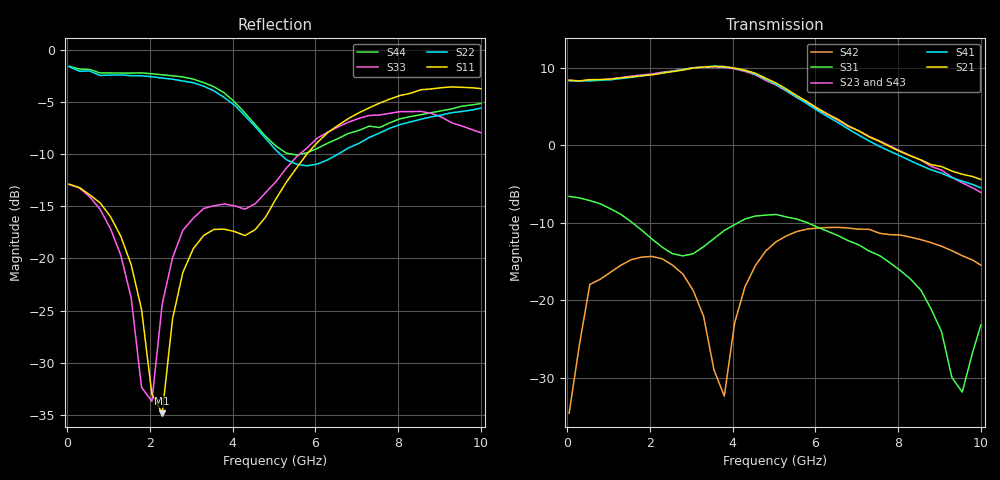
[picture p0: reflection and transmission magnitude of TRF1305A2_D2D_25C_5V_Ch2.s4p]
!Created with skrf (http://scikit-rf.org).
# Hz S MA R 50.0
! PORT[1] = INP
! PORT[2] = OUTM
! PORT[3] = INM
! PORT[4] = OUTP
!freq magS11 angS11 magS12 angS12 magS13 angS13
! magS14 angS14
! magS21 angS21 magS22 angS22 magS23 angS23
! magS24 angS24
! magS31 angS31 magS32 angS32 magS33 angS33
! magS34 angS34
! magS41 angS41 magS42 angS42 magS43 angS43
! magS44 angS44
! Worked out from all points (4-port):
!   41 points, 50 MHz to 10 GHz, reference 50 ohm
!   strongest paths, dB at 50 MHz, 2.55 GHz, 5.05 GHz, 7.55 GHz, 10 GHz:
!     S21: 8.4, 9.5, 8.0, 0.5, -4.4
!     S41: 8.3, 9.5, 7.8, -0.2, -5.5
!     S23: 8.4, 9.6, 7.7, 0.5, -6.1
!     S43: 8.3, 9.5, 7.7, 0.4, -5.9
!     S31: -6.6, -14.0, -9.0, -14.3, -23.2
!     S42: -34.6, -15.5, -12.5, -11.4, -15.5
!   lowest |S11| = -34.8 dB at 2.3 GHz (marker M1), VSWR 1.04, Z = 51.2 + j1.41 ohm
!   |S11| at or under -10 dB: start of sweep to 5.795 GHz
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5e7  0.2266 -3.3  0.00462 54.8  0.4625 -2.6  0.003948 133.1
     2.618 177.2  0.8278 177.5  2.617 -2.4  0.02086 122.0
     0.4668 -3.0  0.004925 134.3  0.2257 -2.3  0.005425 -2.4
     2.593 -2.6  0.01859 127.6  2.592 177.6  0.8326 177.6
2.3e9  0.0181 49.3  0.04119 -35.9  0.2165 -129.9  0.02643 -63.0
       2.911 63.0  0.7302 101.4  2.951 -117.4  0.183 -16.7
       0.2193 -128.6  0.02765 -64.5  0.06053 75.2  0.03866 -33.2
       2.923 -114.5  0.1845 -15.0  2.911 62.3  0.7569 99.3
3.55e9  0.1376 27.0  0.05256 -79.4  0.2484 114.8  0.02407 -130.3
        3.215 -11.6  0.6344 59.3  3.189 166.5  0.0283 -111.0
        0.2491 116.3  0.02722 -131.9  0.1786 35.4  0.05021 -79.5
        3.228 170.3  0.0355 -93.2  3.17 -13.3  0.6632 57.2
4.55e9  0.1375 30.0  0.05845 -120.0  0.3406 56.4  0.01795 -175.7
        2.906 -78.4  0.4267 32.8  2.838 98.9  0.1819 65.6
        0.3484 58.4  0.02007 172.8  0.1828 34.1  0.05493 -122.4
        2.868 103.3  0.1667 70.0  2.82 -80.4  0.4362 32.7
5.8e9  0.3172 22.9  0.05704 -169.0  0.3059 11.5  0.008715 164.8
       1.908 -153.5  0.2776 41.7  1.873 23.7  0.2854 13.9
       0.3163 11.6  0.01159 136.3  0.3383 22.6  0.05504 -172.7
       1.848 27.7  0.2872 18.5  1.863 -154.8  0.3203 42.9
7.55e9  0.5537 -26.5  0.0545 133.1  0.1891 -15.6  0.01148 134.6
        1.055 125.0  0.3983 39.4  1.064 -62.8  0.2544 -25.5
        0.1938 -18.0  0.01113 121.5  0.486 -33.9  0.05486 129.4
        0.98 -54.4  0.2698 -25.0  1.05 122.2  0.4233 33.1
1e10  0.6495 -102.2  0.05077 44.6  0.06623 77.8  0.01433 19.5
      0.5997 26.7  0.5242 1.2  0.4946 -175.5  0.169 -65.1
      0.06911 77.1  0.01509 5.9  0.3995 -148.0  0.04564 24.9
      0.5297 -155.2  0.1678 -64.5  0.508 14.2  0.5512 0.4
